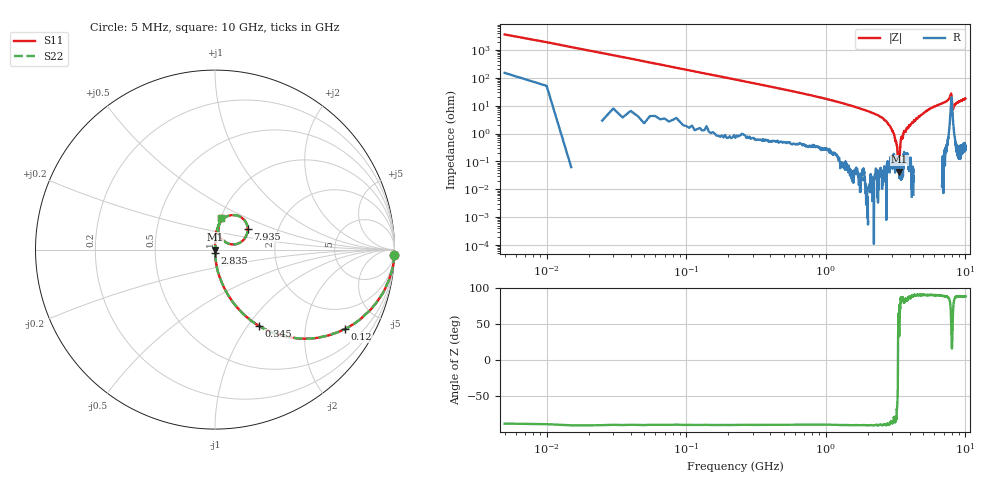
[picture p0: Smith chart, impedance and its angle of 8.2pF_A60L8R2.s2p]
! Amotech Co.,Ltd.
! http://www.amotech.co.kr/
! Part Number: A60L8R2
! These Parameters are Measured in Series Mode Connection
! Operation Temp=25[degC], DC Bias Voltage=0[V]
! Freq. Start=5[MHz] Stop=10[GHz], 2000[Steps]
! Date: Monday, July 14, 2020, 09:34:51
# GHZ S RI R 50.000000
!Freq.(Hz) S11(Real) S11(Imag) S21(Real) S21(Imag) S12(Real) S12(Imag) S22(Real) S22(Imag)
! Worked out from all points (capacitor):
!   2000 points, 5 MHz to 10 GHz, reference 50 ohm
!   read as one part in series: C = 8.13 pF near 55 MHz
!   lowest |Z| = 43.2 mohm at 3.355 GHz (marker M1)
!   series resonance near 3.29 GHz, so ESL is about 290 pH
!   S11 on the Smith chart (normalised r, x): 5 MHz: 4, -72; 120 MHz: 1.03, -3.26; 345 MHz: 1.01, -1.13; 2.835 GHz: 1.00, -0.04; 7.935 GHz: 1.40, +0.34; 10 GHz: 1.01, +0.36
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0.005  0.9981 -0.0276  0.00192 0.0276  0.00192 0.0276  0.9981 -0.0276
0.065  0.899 -0.296  0.101 0.296  0.101 0.296  0.899 -0.296
0.12  0.7243 -0.4424  0.2757 0.4424  0.2757 0.4424  0.7243 -0.4424
0.345  0.2454 -0.4251  0.7546 0.4251  0.7546 0.4251  0.2454 -0.4251
0.73  0.0644 -0.2385  0.9356 0.2385  0.9356 0.2385  0.0644 -0.2385
1.675  0.00781 -0.085  0.9922 0.085  0.9922 0.085  0.00781 -0.085
2.53  0.0015 -0.0374  0.9985 0.0374  0.9985 0.0374  0.0015 -0.0374
2.835  0.00089 -0.0205  0.9991 0.0205  0.9991 0.0205  0.00089 -0.0205
3.055  0.00142 -0.0103  0.9986 0.0103  0.9986 0.0103  0.00142 -0.0103
3.2  0.000947 -0.0044  0.9991 0.0044  0.9991 0.0044  0.000947 -0.0044
3.315  0.000623 0.000704  0.9994 -0.000704  0.9994 -0.000704  0.000623 0.000704
3.34  0.000492 0.00097  0.9995 -0.00097  0.9995 -0.00097  0.000492 0.00097
3.355  0.000359 0.000239  0.9996 -0.000239  0.9996 -0.000239  0.000359 0.000239
3.455  0.000546 0.00646  0.9995 -0.00646  0.9995 -0.00646  0.000546 0.00646
3.645  0.00225 0.0122  0.9977 -0.0122  0.9977 -0.0122  0.00225 0.0122
5.005  0.00185 0.0534  0.9982 -0.0534  0.9982 -0.0534  0.00185 0.0534
6.67  0.0132 0.1149  0.9868 -0.1149  0.9868 -0.1149  0.0132 0.1149
7.625  0.0401 0.1663  0.9599 -0.1663  0.9599 -0.1663  0.0401 0.1663
7.935  0.182 0.1164  0.818 -0.1164  0.818 -0.1164  0.182 0.1164
8.1  0.0483 0.0492  0.9517 -0.0492  0.9517 -0.0492  0.0483 0.0492
8.335  0.0188 0.0984  0.9812 -0.0984  0.9812 -0.0984  0.0188 0.0984
10  0.034 0.1744  0.966 -0.1744  0.966 -0.1744  0.034 0.1744
